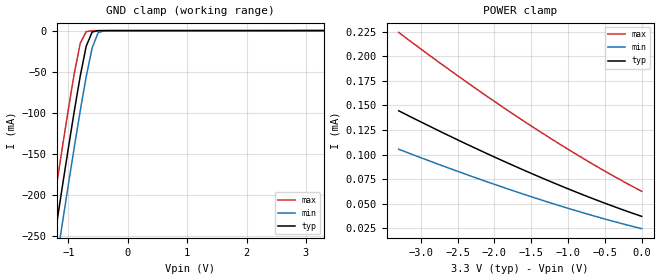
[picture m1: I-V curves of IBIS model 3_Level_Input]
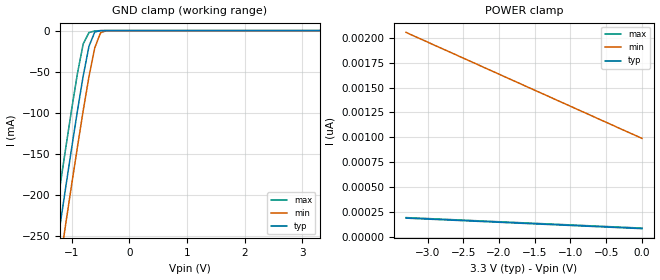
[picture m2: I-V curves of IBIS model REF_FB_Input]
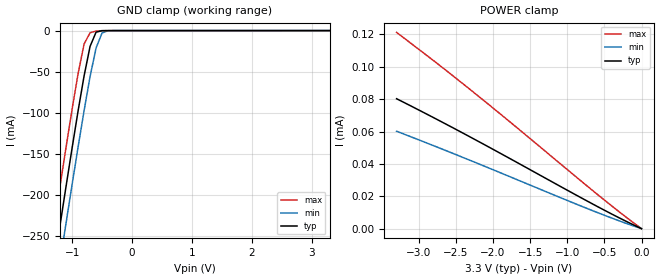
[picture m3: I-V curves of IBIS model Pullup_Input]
| IBIS file qs5v9910.ibs created by s2ibis2 version 1.1
| North Carolina State University Electronics Research Laboratory  1995
[IBIS ver]   2.1
[File name]   qs5v9910.ibs
[File Rev]   1.2
[Date]   Friday, March 17, 2006
[Source]   IDT
[Notes]   1. Temp typ=25C, min=85C, max=-40C 2. QSA 0.8 process 2. Ramp
   rates based on 50 ohm load
[Disclaimer] Integrated Device Technology, Inc. ("IDT") hereby grants the
   user of this IBIS model a non-exclusive, nontransferable
   license to use this IBIS model under the following terms. The
   user is granted this license only to use the IBIS model and is
   not granted rights to sell, copy (except as needed to run the
   IBIS model), rent, lease or sub-license the IBIS model in
   whole or in part, or in modified form to anyone. The User may
   modify the IBIS model to suit its specific applications, but
   rights to derivative works and such modifications shall belong
   to IDT.
   This IBIS model is provided on an "AS IS" basis and IDT
   makes absolutely no warranty with respect to the information
   contained herein. IDT DISCLAIMS AND CUSTOMER WAIVES ALL
   WARRANTIES, EXPRESS AND IMPLIED, INCLUDING WARRANTIES OF
   MERCHANTABILITY AND FITNESS FOR A PARTICULAR PURPOSE. THE
   ENTIRE RISK AS TO QUALITY AND PERFORMANCE IS WITH THE
   USER ACCORDINGLY, IN NO EVENT SHALL IDT BE LIABLE
   FOR ANY DIRECT OR INDIRECT DAMAGES, WHETHER IN CONTRACT OR
   TORT, INCLUDING ANY LOST PROFITS OR OTHER INCIDENTAL,
   CONSEQUENTIAL, EXEMPLARY, OR PUNITIVE DAMAGES ARISING OUT OF
   THE USE OR APPLICATION OF THE IBIS model.  Further, IDT
   reserves the right to make changes without notice to any
   product herein to improve reliability, function, or design.
   IDT does not convey any license under patent rights or
   any other intellectual property rights, including those of
   third parties. IDT is not obligated to provide maintenance
   or support for the licensed IBIS model.
[Copyright]   Copyright 2006, Integrated Device Technology, Inc. all rights
   reserved
|   Component QS5V9910
[Component]   QS5V9910
[Manufacturer]   Integrated Device Technology Inc.
[Package]
|Following package parameters are for 24 pin SOIC package
| variable   typ   min   max
R_pkg   0.40   0.40   0.40
L_pkg   5.70nH   5.70nH   5.70nH
C_pkg   0.40pF   0.40pF   0.40pF
[Pin]  signal_name   model_name   R_pin   L_pin   C_pin
1   REF   REF_FB_Input
2   VCCQ   POWER
4   NC   NC
5   VCCQ/PE   Pullup_Input
6   VCCN   POWER
7   Q0   Output
8   Q1   Output
9   GND   GND
10   Q2   Output
11   Q3   Output
12   VCCN   POWER
13   FB   REF_FB_Input
14   VCCN   POWER
15   Q4   Output
16   Q5   Output
17   GND   GND
18   Q6   Output
19   Q7   Output
21   VCCN   POWER
22   NC   NC
23   TEST   3_Level_Input
24   GND   GND
| Models and submodels in the file (4): 3_Level_Input (Input), REF_FB_Input (Input), Pullup_Input (Input), Output (Output)
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| in   in   dummy_model
|   Model 3_Level_Input
[Model]   3_Level_Input
Model_type   Input
Vinl =  0.80000V
Vinh =  2.00000V
C_comp   5.00000pF   5.00000pF   5.00000pF
[Temperature Range]   25.00000   85.00000   -40.00000
[Voltage Range]   3.30000V   3.00000V   3.60000V
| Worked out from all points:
|   GND clamp passes 1 mA (typ) near -0.56 V on its own axis
[GND_clamp]
| voltage   I(typ)   I(min)   I(max)
-3.3V     -1.264A    -1.307A    -1.219A
-1.4V     -331.8mA   -376.4mA   -284.1mA
-1.3V     -283.8mA   -328.5mA   -236mA
-1.2V     -236.2mA   -281mA     -188.3mA
-1.1V     -189mA     -233.8mA   -141.3mA
-900mV    -97.59mA   -141.5mA   -51.75mA
-800mV    -55.03mA   -97.33mA   -15.18mA
-700mV    -18.94mA   -55.9mA    -1.21mA
-600mV    -1.672mA   -21.04mA   -162.4uA
-500mV    -67.1uA    -2.735mA   -14.13uA
-400mV    -2.461uA   -131.4uA   -334nA
3.3V      36.98uA    30.19uA    51.08uA
[POWER_clamp]
| voltage   I(typ)   I(min)   I(max)
-3.3V     144.6uA    105.4uA    224.5uA
-2.4V     111.4uA    80.19uA    175.1uA
-1.5V     80.8uA     57uA       129.1uA
-700mV    56.12uA    38.52uA    91.83uA
0V        36.98uA    24.41uA    62.51uA
|   Model REF_FB_Input
[Model]   REF_FB_Input
Model_type   Input
Vinl =  0.80000V
Vinh =  2.00000V
C_comp   5.00000pF   5.00000pF   5.00000pF
[Temperature Range]   25.00000   85.00000   -40.00000
[Voltage Range]   3.30000V   3.00000V   3.60000V
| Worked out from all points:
|   GND clamp passes 1 mA (typ) near -0.55 V on its own axis
[GND_clamp]
| voltage   I(typ)   I(min)   I(max)
-3.3V     -1.264A    -1.307A    -1.219A
-1.4V     -331.8mA   -376.4mA   -284.2mA
-1.3V     -283.8mA   -328.5mA   -236.1mA
-1.2V     -236.2mA   -281mA     -188.5mA
-1.1V     -189.1mA   -233.8mA   -141.5mA
-900mV    -97.66mA   -141.6mA   -52.18mA
-800mV    -55.12mA   -97.34mA   -16.15mA
-700mV    -19.08mA   -55.92mA   -2.372mA
-600mV    -1.792mA   -21.05mA   -466.4uA
-500mV    -89uA      -2.742mA   -33.11uA
-400mV    -3.691uA   -131.6uA   -667.8nA
3.3V      81.1pA     1.086nA    77.06pA
[POWER_clamp]
| voltage   I(typ)   I(min)   I(max)
-3.3V     187pA      2.056nA    192.5pA
-2.9V     174.1pA    1.926nA    179.7pA
-2.6V     164.5pA    1.83nA     170.1pA
0V        81.1pA     989.5pA    86.68pA
|   Model Pullup_Input
[Model]   Pullup_Input
Model_type   Input
Vinl =  0.80000V
Vinh =  2.00000V
C_comp   5.00000pF   5.00000pF   5.00000pF
[Temperature Range]   25.00000   85.00000   -40.00000
[Voltage Range]   3.30000V   3.00000V   3.60000V
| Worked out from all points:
|   GND clamp passes 1 mA (typ) near -0.55 V on its own axis
[GND_clamp]
| voltage   I(typ)   I(min)   I(max)
-3.3V     -1.264A    -1.307A    -1.219A
-1.4V     -331.8mA   -376.5mA   -284.3mA
-1.3V     -283.8mA   -328.6mA   -236.2mA
-1.2V     -236.2mA   -281mA     -188.5mA
-1.1V     -189.1mA   -233.8mA   -141.5mA
-900mV    -97.69mA   -141.6mA   -52.25mA
-800mV    -55.17mA   -97.39mA   -16.31mA
-700mV    -19.18mA   -55.98mA   -2.61mA
-600mV    -1.934mA   -21.16mA   -606.1uA
-500mV    -149.3uA   -2.886mA   -87.57uA
-400mV    -30.57uA   -195uA     -42.14uA
3.3V      161.8pA    4.819uA    -9.329uA
[POWER_clamp]
| voltage   I(typ)   I(min)   I(max)
-3.3V     80.31uA    60.21uA    121.3uA
-2.3V     56.45uA    42.05uA    85.67uA
-600mV    13.82uA    10.06uA    21.38uA
0V        161.8pA    1.984nA    172.3pA
